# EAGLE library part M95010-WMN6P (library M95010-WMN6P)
M95010-WMN6P, Serial EEPROM Memory 1kbit, Serial-SPI, 35ns 2.5 5.5 V, 8-Pin SOIC Source: Datasheet
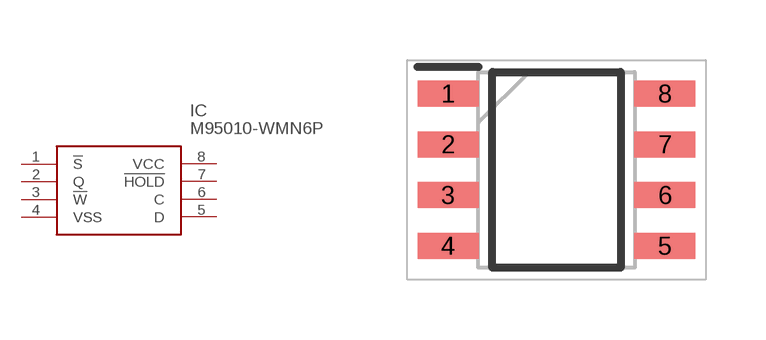
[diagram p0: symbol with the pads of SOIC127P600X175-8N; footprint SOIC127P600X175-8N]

Designator prefix IC

## M95010-WMN6P (Allied_Number: 70389563; Allied_Price-Stock: http://www.alliedelec.com/stmicroelectronics-m95010-wmn6p/70389563/; Description: M95010-WMN6P, Serial EEPROM Memory 1kbit, Serial-SPI, 35ns 2.5 5.5 V, 8-Pin SOIC; Height: 1.75mm; Manufacturer_Name: STMicroelectronics; Manufacturer_Part_Number: M95010-WMN6P; Mouser_Part_Number: 511-M95010-WMN6P; Mouser_Price-Stock: https://www.mouser.com/Search/Refine.aspx?Keyword=511-M95010-WMN6P; RS_Part_Number: 7147617; RS_Price-Stock: http://uk.rs-online.com/web/p/eeprom-memory-chips/7147617/?source=DS)  [SOIC127P600X175-8N]
1  !S
2  Q  out
3  !W
4  VSS  pwr
5  D  in
6  C
7  !HOLD
8  VCC  pwr

## Footprint SOIC127P600X175-8N (pad centres in mm)
SO8 (150 mils width)
smd 1.525 x 0.65: 1 -2.712,1.905; 2 -2.712,0.635; 3 -2.712,-0.635; 4 -2.712,-1.905; 5 2.712,-1.905; 6 2.712,-0.635; 7 2.712,0.635; 8 2.712,1.905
